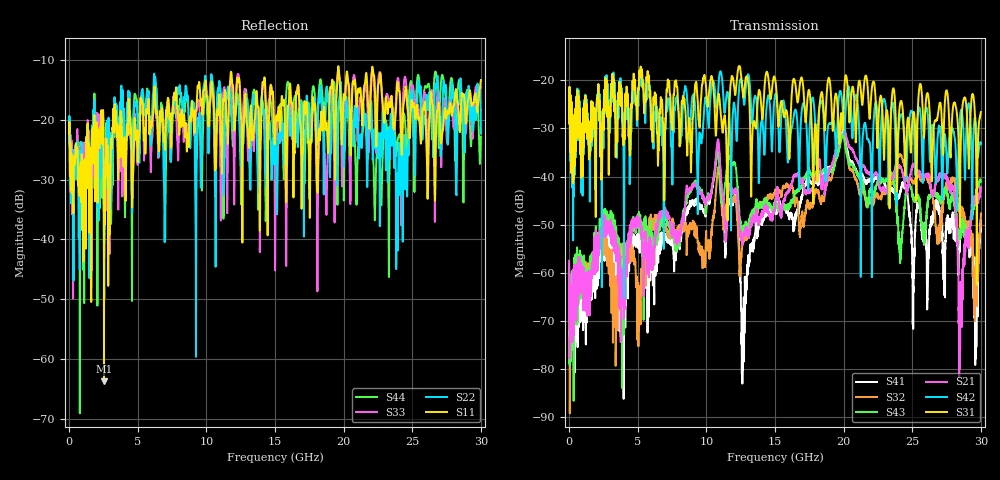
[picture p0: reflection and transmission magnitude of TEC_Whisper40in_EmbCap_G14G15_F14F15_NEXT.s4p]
! Tyco Electronics
! F14F15-G14G15_NEXT
!! PART DESCRIPTION: Whisper 40in Megtron 6 VLP-HVLP-VLP Channel, Embedded Capactior Connecter at one end, bulkhead 2.4mm test pts
!! MODEL DESCRIPTION: System 4-port S-parameter
!! MODEL STATUS: Measured
!! MODEL GEOMETRY: Channel Model
!! MODEL FREQUENCY RANGE: DC to 30.000 GHz in 10.000 MHz frequency steps
!! MODEL EDGE RATE LIMITATION: 12.500 ps (Using conservative 0.5/Fmax rule of thumb)
!! TIME-DOMAIN TRANSFORM CAUTIONS:
!! 1.) Do not simulate transient edge rates faster than the number listed above.  Edge rates faster than this number
!!  contain significant spectral content at frequencies above the model's highest frequency.
!! 2.) Even when simulating edge rates that are slower than the number listed above, be aware that the best time
!!  resolution possible with a direct iFFT is (1 / 2Fmax).  As a result, time resolution is typically not adequate
!!  for most time-domain simulations unless tricks such as windowing are used to minimize leakage and aliasing.
!! 3.) Because the model has a uniform frequency step, a direct iFFT will result in an impulse that that has a time
!!  length given by either (1 / Fstep) or (1 / 2Fstep), depending on the transform being used.  Care has been taken
!!  in selecting the frequency step to ensure a settled impulse response for the model.  Therefore, convolution with
!!  the model's impulse response should present no issues.  However, if directly concatenating s-parameter models
!!  in the frequency domain a user must either interpolate necessary interim frequencies or complete impulse response
!!  zero-padding.  Impulse response zero-padding is more difficult, but more accurate.
!! PORT DEFINITIONS:
!! Port  1  ----->  Side A  F14  G14  Side A  <-----  Port  2
!! Port  3  ----->  Side A  F15  G15  Side A  <-----  Port  4
! Point-to-Point link (differential)  !
! Connectors:  !
!  1: STRADA Whisper  !
! Materials:  !
!  Backplane: Megtron-6 HVLP  !
!  Daughtercard: Megtron-6 VLP  !
! Stack-up:  !
!  Backplane: 20 layers, 200mil thick  !
!  Daughtercard: 14 layers, 110mil thick  !
! Trace Length:  !
!  Backplane: 30in  !
!  Daightercards: 5in  !
! Trace Width:  !
!  Backplane: 7-9-7 mils  !
!  Daughtercards: 6-9-6 mils  !
! Geometry:  !
!  Backplane: Stripline  !
!  Daughtercards: Stripline  !
! Freq. Range: 0 GHz - 30 GHz  !
! Note1: non-mixed-mode s-parameters  !
! Note2: channel includes 2.4mm test points  !
! Touchstone data
! Created: 02-Jul-2013 by IdEM R2011 (7.0.3)
# Hz S MA R 50
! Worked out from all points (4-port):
!   3000 points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, 10 MHz to 30 GHz, reference 50 ohm
!   strongest paths, dB at 10 MHz, 7.51 GHz, 15.01 GHz, 22.51 GHz, 30 GHz:
!     S31: -29.0, -29.2, -19.6, -30.8, -26.6
!     S42: -28.3, -38.4, -23.0, -28.8, -33.2
!     S21: -57.5, -52.5, -45.9, -40.1, -42.3
!     S43: -58.1, -51.3, -45.5, -40.9, -41.1
!     S32: -71.6, -50.0, -43.4, -43.6, -47.7
!     S41: -63.3, -52.9, -47.4, -40.2, -49.4
!   lowest |S11| = -63.8 dB at 2.55 GHz (marker M1), VSWR 1.00, Z = 50 - j0.0522 ohm
!   |S11| at or under -10 dB: start of sweep to end of sweep
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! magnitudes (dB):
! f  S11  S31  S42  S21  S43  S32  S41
! 10 MHz  -22.2  -29.0  -28.3  -57.5  -58.1  -71.6  -63.3
! 2.55 GHz  -63.8  -24.2  -22.5  -48.4  -47.4  -51.5  -51.2
! 10.84 GHz  -19.1  -24.4  -23.6  -32.4  -35.0  -38.6  -33.0
! 12.67 GHz  -23.3  -23.0  -22.8  -52.7  -50.9  -53.0  -73.1
! 19.97 GHz  -17.5  -28.9  -27.9  -29.1  -31.5  -31.1  -30.6
! 28.52 GHz  -19.5  -35.3  -26.6  -61.9  -51.4  -46.1  -51.8
! 30 GHz  -13.3  -26.6  -33.2  -42.3  -41.1  -47.7  -49.4
